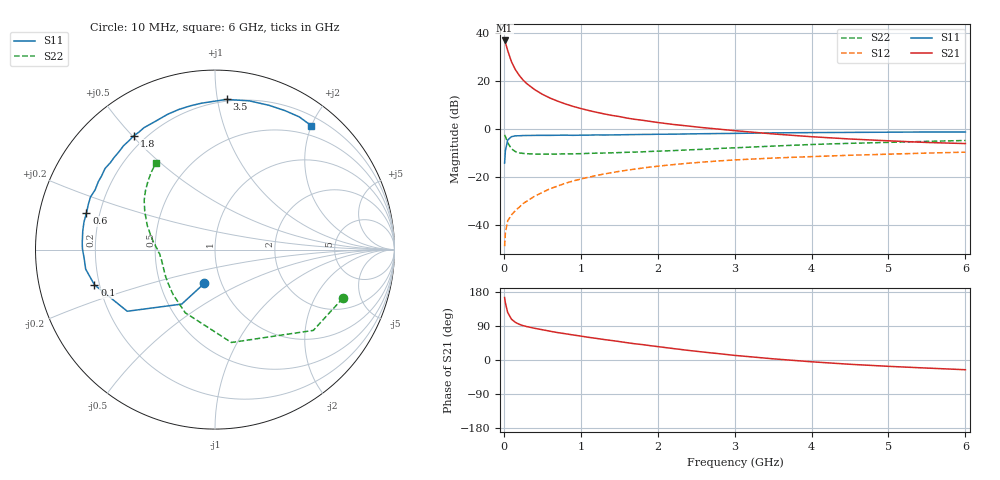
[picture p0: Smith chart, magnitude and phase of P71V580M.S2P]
! SIEMENS Small Signal Semiconductors
! BFP196
! Si NPN RF Bipolar Junction Transistor in SOT143
! VCE = 1.5 V  IC = 80 mA
! Common Emitter S-Parameters:  May  1996
# GHz  S  MA  R  50
!  f  S11  S21  S12  S22
! GHz  MAG  ANG  MAG  ANG  MAG  ANG  MAG  ANG
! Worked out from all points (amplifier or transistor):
!   36 points, 10 MHz to 6 GHz, reference 50 ohm
!   highest |S21| = 36.9 dB at 10 MHz (marker M1)
!   |S21| within 3 dB of that: start of sweep to 39.16 MHz
!   unconditionally stable (mu >= 1): 292.8 MHz to 5.414 GHz; 5.625 GHz to end of sweep
!   at 250 MHz: K = 0.96, MSG = 25.7 dB, |S12| = -30.9 dB
!   at 1.4 GHz: K = 1.12, MAG = 9.9 dB, |S12| = -18.1 dB
!   at 6 GHz: K = 1.01, MAG = 1.3 dB, |S12| = -9.5 dB
!   S11 on the Smith chart (normalised r, x): 10 MHz: 0.83, -0.33; 100 MHz: 0.18, -0.14; 600 MHz: 0.15, +0.14; 1.8 GHz: 0.16, +0.51; 3.5 GHz: 0.19, +1.06; 6 GHz: 0.34, +1.99
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0.01  0.1977 -107.6  70.06 164.9  0.0037 71.9  0.7616 -20.9
0.02  0.3556 -121.4  63.43 150.7  0.007 67.1  0.7091 -39.4
0.05  0.5974 -144.9  43.15 125.3  0.0124 52.4  0.5255 -80.0
0.1  0.6996 -163.7  25.11 107.5  0.0166 51.1  0.3888 -115.3
0.15  0.7287 -171.4  17.33 99.3  0.0203 53.5  0.3427 -132.9
0.2  0.7309 -176.4  13.17 94.2  0.0239 57.8  0.323 -143.4
0.25  0.7385 179.7  10.53 90.7  0.0284 60.2  0.3138 -150.9
0.3  0.7406 177.1  8.821 88.1  0.032 62.2  0.3091 -155.2
0.4  0.7441 171.9  6.664 83.7  0.0404 64.8  0.3043 -161.8
0.5  0.746 168.1  5.333 79.9  0.0484 65.7  0.3032 -166.0
0.6  0.7448 164.1  4.448 76.0  0.0578 65.9  0.3036 -168.9
0.7  0.7496 160.2  3.831 72.3  0.0659 65.8  0.3049 -171.1
0.8  0.753 157.1  3.356 69.3  0.0752 64.7  0.3068 -172.9
1.1  0.7534 147.0  2.458 59.9  0.1005 61.7  0.3146 -177.4
1.4  0.7611 137.6  1.944 51.5  0.1246 57.4  0.3229 179.0
1.8  0.7791 125.5  1.537 40.7  0.1556 51.2  0.3386 174.5
2.2  0.7882 114.8  1.258 30.3  0.1834 44.9  0.359 169.4
2.8  0.8127 99.7  1.002 16.6  0.2195 35.6  0.3982 160.9
3.5  0.8394 85.6  0.798 3.1  0.2513 25.3  0.4459 151.4
4.5  0.8584 69.5  0.626 -11.3  0.2873 13.1  0.5089 139.5
5.5  0.8759 57.6  0.53 -21.3  0.3188 2.2  0.5593 129.4
6  0.8743 52.2  0.503 -25.7  0.3333 -3.5  0.5829 124.4
